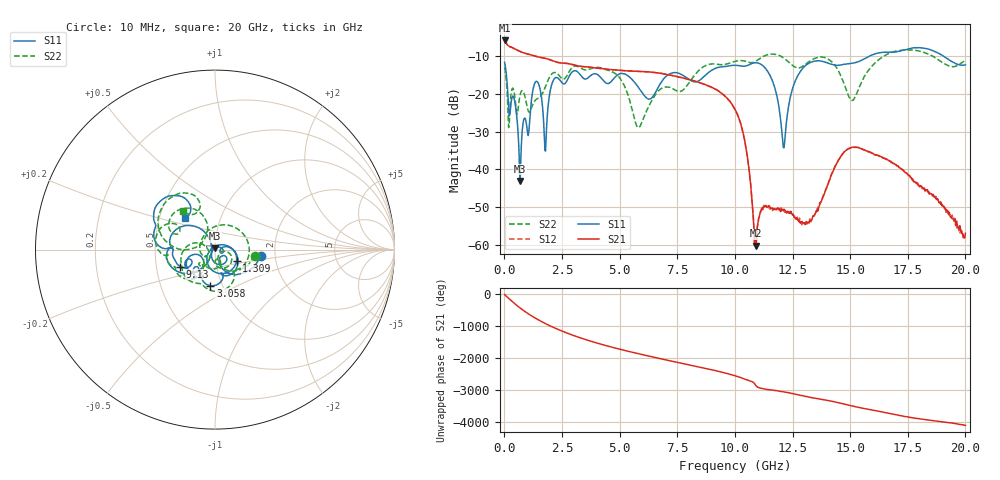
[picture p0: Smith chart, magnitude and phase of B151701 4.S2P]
!  2-Port S-parameters saved by WinCal
! VAR MeasName=S-Parameters (CALIBRATED_DATA) read from VNA (N5244A)
! VAR MeasDate=2015-12-24 19:08:39
! VAR NAME=B151701 4
! VAR FILENAME=B151701 4.S2P
! VAR DATE=2015-12-24 19:08:39
! VAR PHYS_PORTS=1,3
# Hz S DB R 50
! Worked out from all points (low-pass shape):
!   801 points, 10 MHz to 20 GHz, reference 50 ohm
!   highest |S21| = -5.88 dB at 10 MHz (marker M1); lowest = -60.3 dB at 10.9 GHz (marker M2)
!   |S21| within 3 dB of the highest: start of sweep to 713.9 MHz
!   lowest |S11| = -43.1 dB at 684.7 MHz (marker M3), VSWR 1.01, Z = 49.8 + j0.656 ohm
!   |S11| at or under -10 dB: start of sweep to 15.85 GHz; 19.04 GHz to end of sweep
!   |S22| runs from -29.0 to -8.4 dB; largest |S21 - S12| = 0.0011
!   S11 on the Smith chart (normalised r, x): 10 MHz: 1.69, -0.12; 1.309 GHz: 1.26, -0.16; 3.058 GHz: 0.88, -0.37; 9.13 GHz: 0.67, -0.13; 20 GHz: 0.68, +0.25
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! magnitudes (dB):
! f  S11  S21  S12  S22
! 10 MHz  -11.7  -5.9  -5.9  -13.0
! 209.9 MHz  -25.9  -7.4  -7.4  -28.6
! 684.7 MHz  -43.1  -8.8  -8.8  -20.3
! 1.309 GHz  -17.3  -10.0  -10.0  -22.0
! 1.784 GHz  -35.2  -10.6  -10.6  -18.1
! 2.134 GHz  -16.3  -11.4  -11.4  -14.4
! 3.058 GHz  -13.9  -12.4  -12.4  -12.7
! 3.358 GHz  -15.5  -12.8  -12.8  -13.3
! 4.908 GHz  -15.0  -13.8  -13.8  -15.1
! 5.807 GHz  -18.2  -14.1  -14.1  -29.0
! 6.682 GHz  -18.2  -14.5  -14.5  -19.3
! 9.13 GHz  -13.3  -18.7  -18.7  -12.1
! 10.01 GHz  -12.5  -24.1  -24.1  -11.4
! 10.48 GHz  -12.6  -34.3  -34.3  -11.4
! 10.9 GHz  -11.8  -60.3  -59.8  -11.4
! 11.65 GHz  -17.0  -50.6  -50.4  -9.5
! 12.1 GHz  -34.3  -50.6  -51.0  -10.5
! 12.6 GHz  -16.9  -52.7  -52.8  -12.9
! 13.35 GHz  -11.5  -53.1  -52.8  -11.0
! 15.1 GHz  -11.9  -34.1  -34.2  -21.8
! 16.68 GHz  -9.0  -37.7  -37.6  -9.3
! 20 GHz  -12.3  -56.9  -58.9  -11.1
